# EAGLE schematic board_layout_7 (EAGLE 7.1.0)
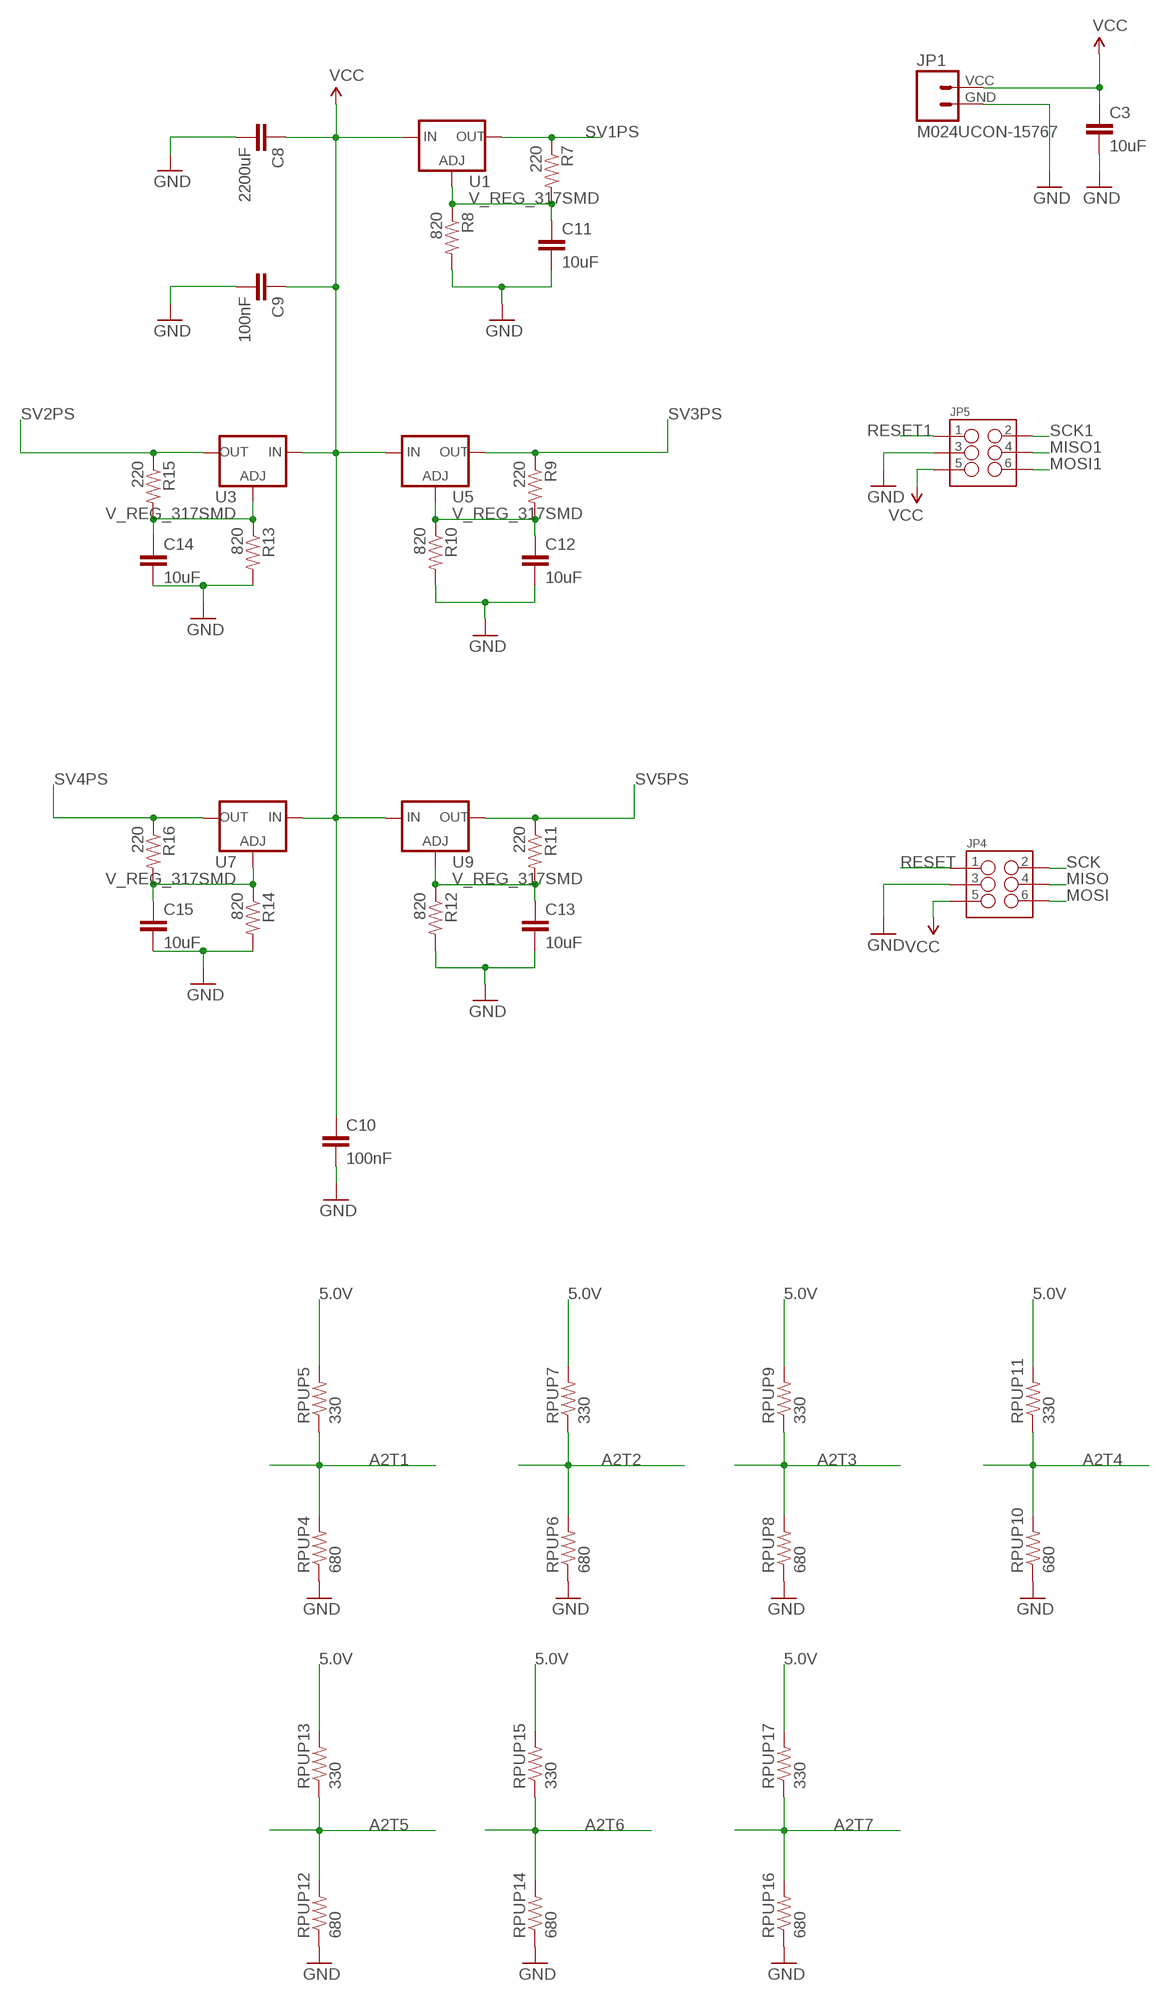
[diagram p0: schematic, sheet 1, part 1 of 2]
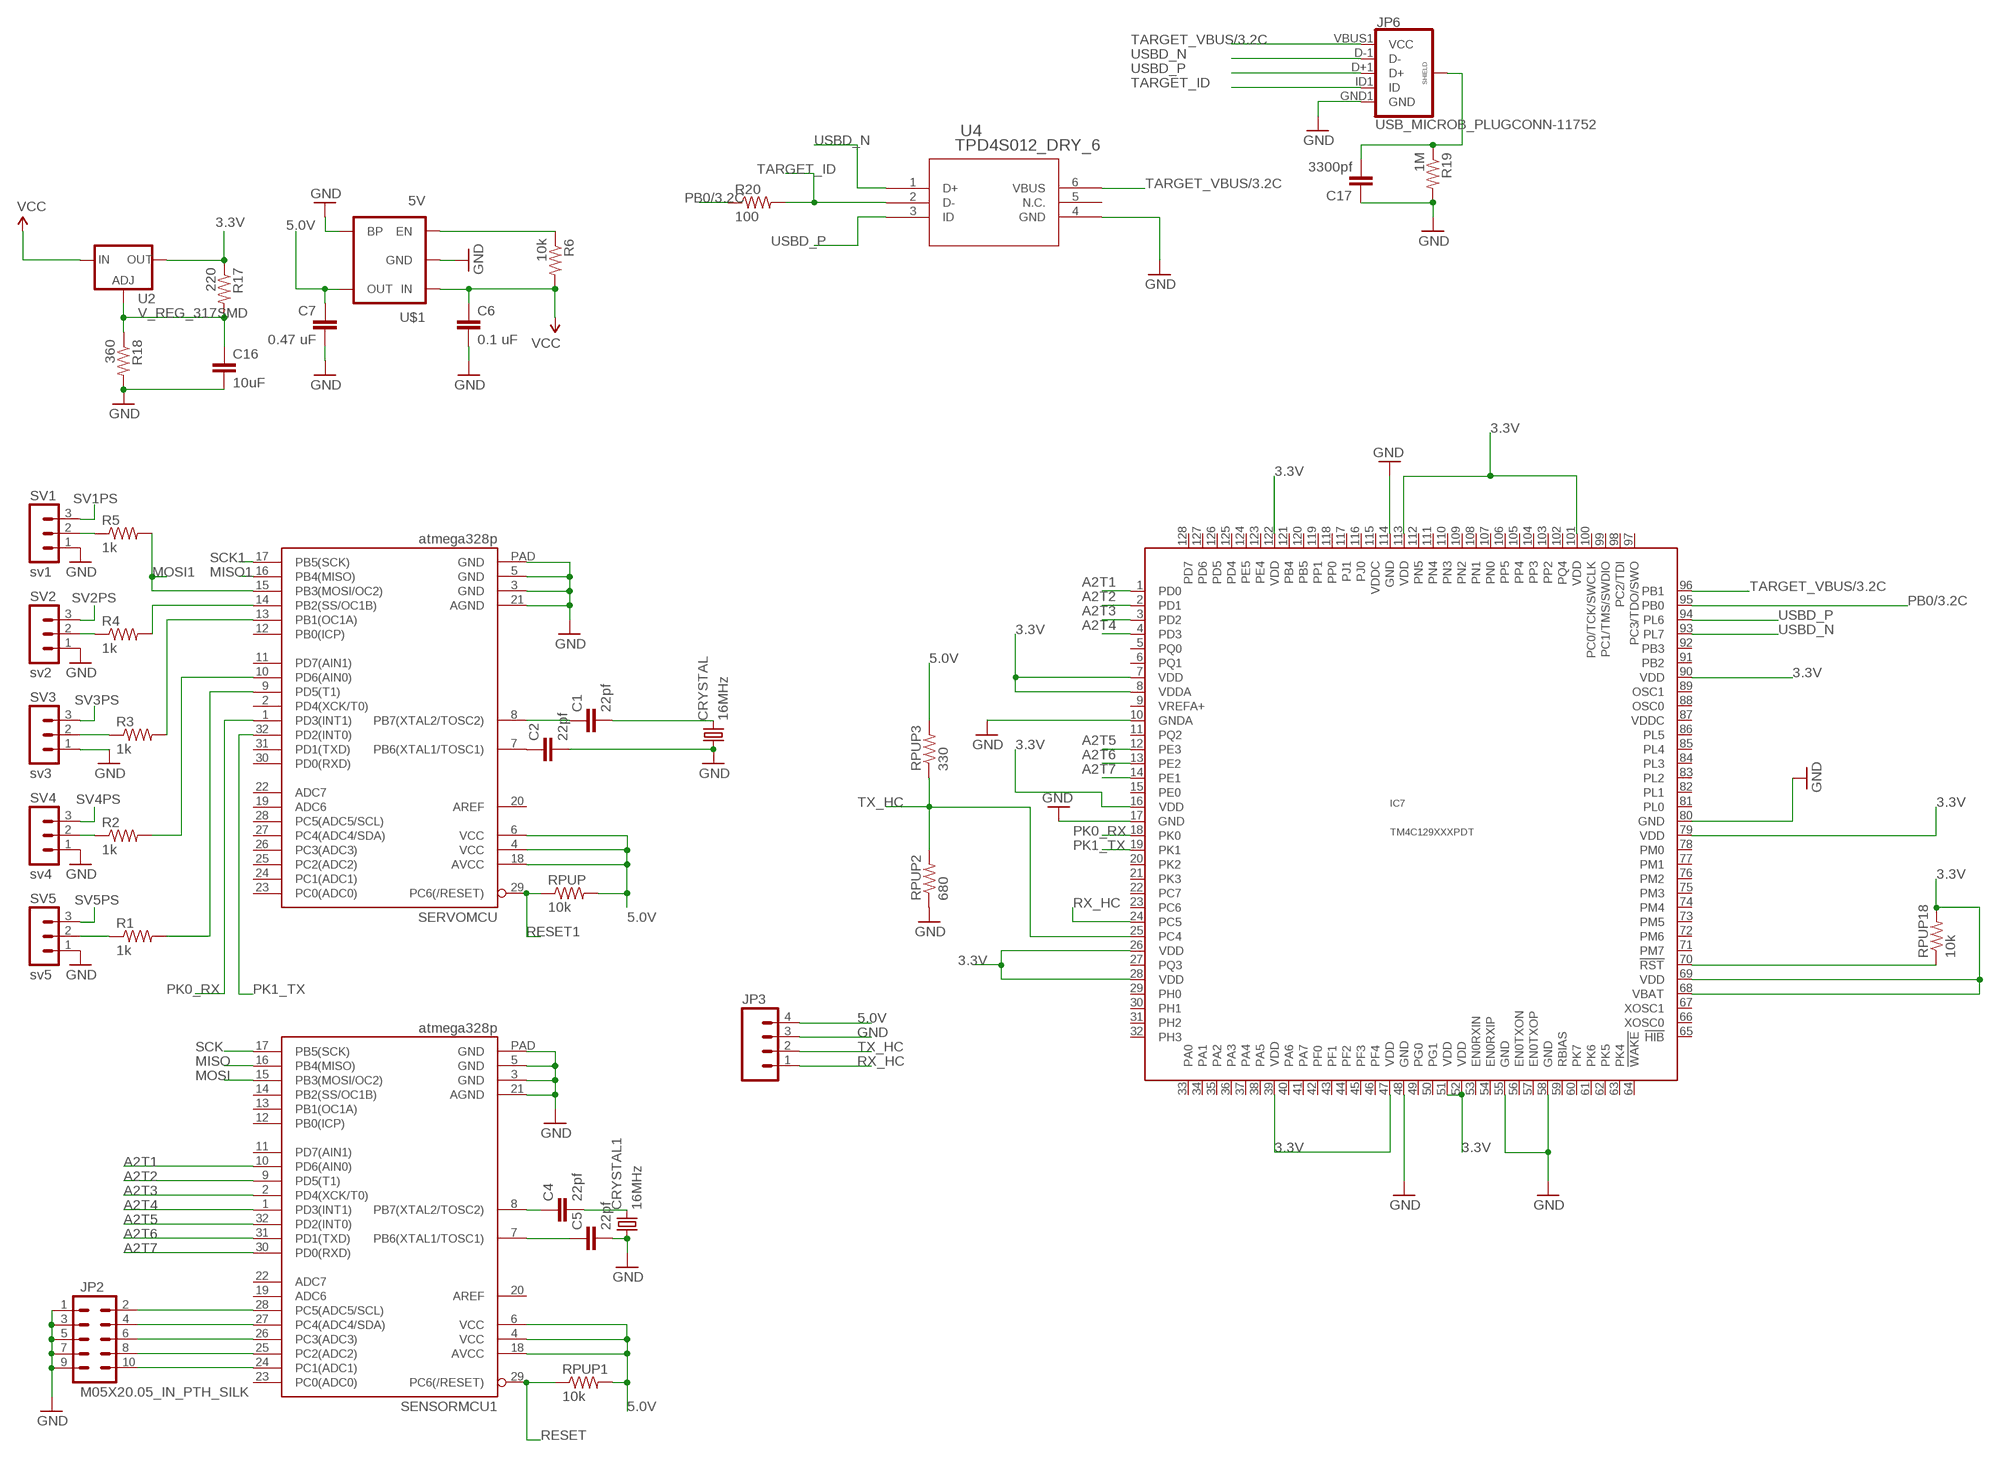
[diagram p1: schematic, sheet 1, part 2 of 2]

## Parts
C1  22pf  CAP0402-CAP  [0402-CAP]
C2  22pf  CAP0402-CAP  [0402-CAP]
C3  10uF  CAP0805  [0805]
C4  22pf  CAP0402-CAP  [0402-CAP]
C5  22pf  CAP0402-CAP  [0402-CAP]
C6  0.1 uF  CAP0805  [0805]
C7  0.47 uF  CAP0805  [0805]
C8  2200uF  CAP0805  [0805]
C9  100nF  CAP0805  [0805]
C10  100nF  CAP0805  [0805]
C11  10uF  CAP0805  [0805]
C12  10uF  CAP0805  [0805]
C13  10uF  CAP0805  [0805]
C14  10uF  CAP0805  [0805]
C15  10uF  CAP0805  [0805]
C16  10uF  CAP0805  [0805]
C17  3300pf  CAP0402-CAP  [0402-CAP]
CRYSTAL  16MHz  CRYSTALTC26V  [TC26V]
CRYSTAL1  16MHz  CRYSTALTC26V  [TC26V]
IC7  TM4C129XXXPDT  [PDT_S-PQFP-G128]
JP1  M024UCON-15767  [JST-2-SMD-VERT]
JP2  M05X20.05_IN_PTH_SILK  [2X5_PTH_SILK_.05]
JP3  M04SMD  [1X04-SMD]
JP4  M03X2  [2X3_SMD]
JP5  M03X2  [2X3_SMD]
JP6  USB_MICROB_PLUGCONN-11752  [USB-B-MICRO-SMD_V03]
R1  1k  RESISTOR0402-RES  [0402-RES]
R2  1k  RESISTOR0402-RES  [0402-RES]
R3  1k  RESISTOR0402-RES  [0402-RES]
R4  1k  RESISTOR0402-RES  [0402-RES]
R5  1k  RESISTOR0402-RES  [0402-RES]
R6  10k  RESISTOR0805-RES  [0805]
R7  220  RESISTOR0805-RES  [0805]
R8  820  RESISTOR0805-RES  [0805]
R9  220  RESISTOR0805-RES  [0805]
R10  820  RESISTOR0805-RES  [0805]
R11  220  RESISTOR0805-RES  [0805]
R12  820  RESISTOR0805-RES  [0805]
R13  820  RESISTOR0805-RES  [0805]
R14  820  RESISTOR0805-RES  [0805]
R15  220  RESISTOR0805-RES  [0805]
R16  220  RESISTOR0805-RES  [0805]
R17  220  RESISTOR0805-RES  [0805]
R18  360  RESISTOR0805-RES  [0805]
R19  1M  RESISTOR0805-RES  [0805]
R20  100  RESISTOR0805-RES  [0805]
RPUP  10k  RESISTOR0402-RES  [0402-RES]
RPUP1  10k  RESISTOR0402-RES  [0402-RES]
RPUP2  680  RESISTOR0402-RES  [0402-RES]
RPUP3  330  RESISTOR0402-RES  [0402-RES]
RPUP4  680  RESISTOR0402-RES  [0402-RES]
RPUP5  330  RESISTOR0402-RES  [0402-RES]
RPUP6  680  RESISTOR0402-RES  [0402-RES]
RPUP7  330  RESISTOR0402-RES  [0402-RES]
RPUP8  680  RESISTOR0402-RES  [0402-RES]
RPUP9  330  RESISTOR0402-RES  [0402-RES]
RPUP10  680  RESISTOR0402-RES  [0402-RES]
RPUP11  330  RESISTOR0402-RES  [0402-RES]
RPUP12  680  RESISTOR0402-RES  [0402-RES]
RPUP13  330  RESISTOR0402-RES  [0402-RES]
RPUP14  680  RESISTOR0402-RES  [0402-RES]
RPUP15  330  RESISTOR0402-RES  [0402-RES]
RPUP16  680  RESISTOR0402-RES  [0402-RES]
RPUP17  330  RESISTOR0402-RES  [0402-RES]
RPUP18  10k  RESISTOR0402-RES  [0402-RES]
SENSORMCU1  atmega328p  ATMEGA328P_MLFMLF32  [MLF32-PAD]
SERVOMCU  atmega328p  ATMEGA328P_MLFMLF32  [MLF32-PAD]
SV1  sv1  MA03-1  [MA03-1]
SV2  sv2  MA03-1  [MA03-1]
SV3  sv3  MA03-1  [MA03-1]
SV4  sv4  MA03-1  [MA03-1]
SV5  sv5  MA03-1  [MA03-1]
U1  V_REG_317SMD  [SOT223]
U2  V_REG_317SMD  [SOT223]
U3  V_REG_317SMD  [SOT223]
U4  TPD4S012_DRY_6  [DRY6]
U5  V_REG_317SMD  [SOT223]
U7  V_REG_317SMD  [SOT223]
U9  V_REG_317SMD  [SOT223]
U$1  5V  V_REG_MIC52055V  [SOT23-5]

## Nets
3.3V: IC7.7(VDD) IC7.8(VDDA) IC7.16(VDD) IC7.26(VDD) IC7.28(VDD) IC7.39(VDD) IC7.47(VDD) IC7.51(VDD) IC7.52(VDD) IC7.68(VBAT) IC7.69(VDD) IC7.79(VDD) IC7.90(VDD) IC7.101(VDD) IC7.113(VDD) IC7.122(VDD) R17.1 RPUP18.2 U2.2(OUT)
5.0V: C7.1 JP3.4 RPUP1.2 RPUP3.2 RPUP5.2 RPUP7.2 RPUP9.2 RPUP11.2 RPUP13.2 RPUP15.2 RPUP17.2 RPUP.2 SENSORMCU1.4(VCC) SENSORMCU1.6(VCC) SENSORMCU1.18(AVCC) SERVOMCU.4(VCC) SERVOMCU.6(VCC) SERVOMCU.18(AVCC) U$1.5(OUT)
A2T1: IC7.1(PD0) RPUP4.2 RPUP5.1 SENSORMCU1.10(PD6(AIN0))
A2T2: IC7.2(PD1) RPUP6.2 RPUP7.1 SENSORMCU1.9(PD5(T1))
A2T3: IC7.3(PD2) RPUP8.2 RPUP9.1 SENSORMCU1.2(PD4(XCK/T0))
A2T4: IC7.4(PD3) RPUP10.2 RPUP11.1 SENSORMCU1.1(PD3(INT1))
A2T5: IC7.12(PE3) RPUP12.2 RPUP13.1 SENSORMCU1.32(PD2(INT0))
A2T6: IC7.13(PE2) RPUP14.2 RPUP15.1 SENSORMCU1.31(PD1(TXD))
A2T7: IC7.14(PE1) RPUP16.2 RPUP17.1 SENSORMCU1.30(PD0(RXD))
GND: C2.2 C3.2 C5.2 C6.2 C7.2 C8.2 C9.2 C10.2 C11.2 C12.2 C13.2 C14.2 C15.2 C16.2 C17.1 CRYSTAL1.1 CRYSTAL.1 IC7.10(GNDA) IC7.17(GND) IC7.48(GND) IC7.55(GND) IC7.58(GND) IC7.80(GND) IC7.114(GND) JP1.GND JP2.1 JP2.3 JP2.5 JP2.7 JP2.9 JP3.3 JP4.3 JP5.3 JP6.GND1(GND) R8.2 R10.2 R12.2 R13.2 R14.2 R18.2 R19.2 RPUP2.1 RPUP4.1 RPUP6.1 RPUP8.1 RPUP10.1 RPUP12.1 RPUP14.1 RPUP16.1 SENSORMCU1.3(GND) SENSORMCU1.5(GND) SENSORMCU1.21(AGND) SENSORMCU1.PAD(GND) SERVOMCU.3(GND) SERVOMCU.5(GND) SERVOMCU.21(AGND) SERVOMCU.PAD(GND) SV1.1 SV2.1 SV3.1 SV4.1 SV5.1 U4.4(GND) U$1.2(GND) U$1.4(BP)
MISO: JP4.4 SENSORMCU1.16(PB4(MISO))
MISO1: JP5.4 SERVOMCU.16(PB4(MISO))
MOSI: JP4.6 SENSORMCU1.15(PB3(MOSI/OC2))
MOSI1: JP5.6 R5.2 SERVOMCU.15(PB3(MOSI/OC2))
N$1: R6.1 U$1.3(EN)
N$2: R4.2 SERVOMCU.14(PB2(SS/OC1B))
N$3: R3.2 SERVOMCU.13(PB1(OC1A))
N$4: C11.1 R7.2 R8.1 U1.1(ADJ)
N$5: R2.1 SV4.2
N$6: R1.1 SV5.2
N$7: R2.2 SERVOMCU.10(PD6(AIN0))
N$8: R1.2 SERVOMCU.9(PD5(T1))
N$9: R3.1 SV3.2
N$10: C1.1 SERVOMCU.8(PB7(XTAL2/TOSC2))
N$11: C2.1 SERVOMCU.7(PB6(XTAL1/TOSC1))
N$12: R5.1 SV1.2
N$13: R4.1 SV2.2
N$14: C16.1 R17.2 R18.1 U2.1(ADJ)
N$15: JP2.10 SENSORMCU1.24(PC1(ADC1))
N$16: JP2.8 SENSORMCU1.25(PC2(ADC2))
N$17: C4.1 SENSORMCU1.8(PB7(XTAL2/TOSC2))
N$18: C4.2 CRYSTAL1.2
N$19: C5.1 SENSORMCU1.7(PB6(XTAL1/TOSC1))
N$20: C1.2 CRYSTAL.2
N$21: JP2.6 SENSORMCU1.26(PC3(ADC3))
N$22: JP2.4 SENSORMCU1.27(PC4(ADC4/SDA))
N$23: JP2.2 SENSORMCU1.28(PC5(ADC5/SCL))
N$25: C12.1 R9.2 R10.1 U5.1(ADJ)
N$26: C13.1 R11.2 R12.1 U9.1(ADJ)
N$29: C14.1 R13.1 R15.2 U3.1(ADJ)
N$31: C15.1 R14.1 R16.2 U7.1(ADJ)
N$38: C17.2 JP6.SHIELD1(SHIELD) JP6.SHIELD2(SHIELD) JP6.SHIELD3(SHIELD) R19.1
N$41: IC7.70(!RST) RPUP18.1
PB0/3.2C: IC7.95(PB0) R20.1
PK0_RX: IC7.18(PK0) SERVOMCU.1(PD3(INT1))
PK1_TX: IC7.19(PK1) SERVOMCU.32(PD2(INT0))
RESET: JP4.1 RPUP1.1 SENSORMCU1.29(PC6(/RESET))
RESET1: JP5.1 RPUP.1 SERVOMCU.29(PC6(/RESET))
RX_HC: IC7.24(PC5) JP3.1
SCK: JP4.2 SENSORMCU1.17(PB5(SCK))
SCK1: JP5.2 SERVOMCU.17(PB5(SCK))
SV1PS: R7.1 SV1.3 U1.2(OUT)
SV2PS: R15.1 SV2.3 U3.2(OUT)
SV3PS: R9.1 SV3.3 U5.2(OUT)
SV4PS: R16.1 SV4.3 U7.2(OUT)
SV5PS: R11.1 SV5.3 U9.2(OUT)
TARGET_ID: JP6.ID1(ID) R20.2 U4.2(D-)
TARGET_VBUS/3.2C: IC7.96(PB1) JP6.VBUS1(VCC) U4.6(VBUS)
TX_HC: IC7.25(PC4) JP3.2 RPUP2.2 RPUP3.1
USBD_N: IC7.93(PL7) JP6.D-1(D-) U4.1(D+)
USBD_P: IC7.94(PL6) JP6.D+1(D+) U4.3(ID)
VCC: C3.1 C6.1 C8.1 C9.1 C10.1 JP1.VCC JP4.5 JP5.5 R6.2 U1.3(IN) U2.3(IN) U3.3(IN) U5.3(IN) U7.3(IN) U9.3(IN) U$1.1(IN)
Unconnected: IC7.5(PQ0) IC7.6(PQ1) IC7.9(VREFA+) IC7.11(PQ2) IC7.15(PE0) IC7.20(PK2) IC7.21(PK3) IC7.22(PC7) IC7.23(PC6) IC7.27(PQ3) IC7.29(PH0) IC7.30(PH1) IC7.31(PH2) IC7.32(PH3) IC7.33(PA0) IC7.34(PA1) IC7.35(PA2) IC7.36(PA3) IC7.37(PA4) IC7.38(PA5) IC7.40(PA6) IC7.41(PA7) IC7.42(PF0) IC7.43(PF1) IC7.44(PF2) IC7.45(PF3) IC7.46(PF4) IC7.49(PG0) IC7.50(PG1) IC7.53(EN0RXIN) IC7.54(EN0RXIP) IC7.56(EN0TXON) IC7.57(EN0TXOP) IC7.59(RBIAS) IC7.60(PK7) IC7.61(PK6) IC7.62(PK5) IC7.63(PK4) IC7.64(!WAKE) IC7.65(!HIB) IC7.66(XOSC0) IC7.67(XOSC1) IC7.71(PM7) IC7.72(PM6) IC7.73(PM5) IC7.74(PM4) IC7.75(PM3) IC7.76(PM2) IC7.77(PM1) IC7.78(PM0) IC7.81(PL0) IC7.82(PL1) IC7.83(PL2) IC7.84(PL3) IC7.85(PL4) IC7.86(PL5) IC7.87(VDDC) IC7.88(OSC0) IC7.89(OSC1) IC7.91(PB2) IC7.92(PB3) IC7.97(PC3/TDO/SWO) IC7.98(PC2/TDI) IC7.99(PC1/TMS/SWDIO) IC7.100(PC0/TCK/SWCLK) IC7.102(PQ4) IC7.103(PP2) IC7.104(PP3) IC7.105(PP4) IC7.106(PP5) IC7.107(PN0) IC7.108(PN1) IC7.109(PN2) IC7.110(PN3) IC7.111(PN4) IC7.112(PN5) IC7.115(VDDC) IC7.116(PJ0) IC7.117(PJ1) IC7.118(PP0) IC7.119(PP1) IC7.120(PB5) IC7.121(PB4) IC7.123(PE4) IC7.124(PE5) IC7.125(PD4) IC7.126(PD5) IC7.127(PD6) IC7.128(PD7) SENSORMCU1.11(PD7(AIN1)) SENSORMCU1.12(PB0(ICP)) SENSORMCU1.13(PB1(OC1A)) SENSORMCU1.14(PB2(SS/OC1B)) SENSORMCU1.19(ADC6) SENSORMCU1.20(AREF) SENSORMCU1.22(ADC7) SENSORMCU1.23(PC0(ADC0)) SERVOMCU.2(PD4(XCK/T0)) SERVOMCU.11(PD7(AIN1)) SERVOMCU.12(PB0(ICP)) SERVOMCU.19(ADC6) SERVOMCU.20(AREF) SERVOMCU.22(ADC7) SERVOMCU.23(PC0(ADC0)) SERVOMCU.24(PC1(ADC1)) SERVOMCU.25(PC2(ADC2)) SERVOMCU.26(PC3(ADC3)) SERVOMCU.27(PC4(ADC4/SDA)) SERVOMCU.28(PC5(ADC5/SCL)) SERVOMCU.30(PD0(RXD)) SERVOMCU.31(PD1(TXD)) U4.5(N.C.)

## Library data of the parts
C1 C2 C4-C7 C17 = SparkFun-Passives:CAP: Capacitor
C3 C8-C16 = SparkFun-Capacitors:CAP: Capacitor
CRYSTAL CRYSTAL1 = crystal:CRYSTAL: CRYSTAL; OC_FARNELL: unknown; OC_NEWARK: unknown
IC7 = ti-tiva:TM4C129XXX
JP1 = SparkFun-Connectors:M02: Standard 2-pin 0.1" header. Use with
JP2 = SparkFun-Connectors:M05X2: Header 5x2 Standard 10-pin dual row 0.1" header. Commonly used with AVR-ISP. Use with Spark Fun Electronics SKU: PRT-00778
JP3 = SparkFun-Connectors:M04: Header 4 Standard 4-pin 0.1" header. Use with straight break away headers (SKU : PRT-00116), right angle break away headers (PRT-00553), swiss pins (PRT-00743), machine pins (PRT-00117), and female headers (PRT-00115). Molex polarized connector foot print use with SKU : PRT-08231 with associated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
JP4 JP5 = SparkFun-Connectors:M03X2: 2x3 .1" header. Shrouded, with keying- CONN-10681 SMT- CONN-11415 Pogo pins- HW-11044; PROD_ID: CONN-11290
JP6 = SparkFun-Connectors:USB_MICROB_PLUG: USB Micro-B connectors Some male, some female. Watch your step!; PROD_ID: CONN-11752
R1-R20 RPUP RPUP1-RPUP18 = SparkFun-Passives:RESISTOR: Resistor
SENSORMCU1 SERVOMCU = SparkFun-DigitalIC:ATMEGA328P_MLF: 32-Pin Atmega328 part Commonly used on Arduino compatible boards Available in QFP and QFN packages TQFP is IC-09069 QFN is non-stock
SV1-SV5 = con-lstb:MA03-1: PIN HEADER; OC_FARNELL: unknown; OC_NEWARK: unknown
U1-U3 U5 U7 U9 = SparkFun-PowerIC:V_REG_317: Voltage Regulator Standard LM317 adjustable voltage regulator. AOI (Adjust Output Input). Google 'LM317 Calculator' for easy to use app to get the two resistor values needed. 240/720 for 5V output. 240/390 for 3.3V output. Spark Fun Electronics SKU : COM-00527
U4 = esd_tp:TPD4S012_DRY_6; DATASHEETURL: http://www.ti.com/lit/gpn/TPD4S012; DESCRIPTION: 4-Channel USB ESD Solution with Power Clamp; FAMILY_NAME: ESD Solution; GENERIC_PART_NUMBER: TPD4S012; INDUSTRY_STD_PKG_TYPE: SON; MANUFACTURER: Texas Instruments; MANUFACTURER_PART_NUMBER: tpd4s012_dry_6; PACKAGE_DESIGNATOR: DRY; PIN_COUNT: 6; VENDOR: Texas Instruments
U$1 = SparkFun-PowerIC:V_REG_MIC5205: V_REG MIC5219 Standard 3.3V and 5V 150mA LDO voltage regulator in SOT-23 layout. Micrel part MIC5205. BP (by-pass) pin is used to lower output noise with 470pF cap, may be left open.; PROD_ID: VREG-00823

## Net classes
0 default: clearance 0.205 mm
